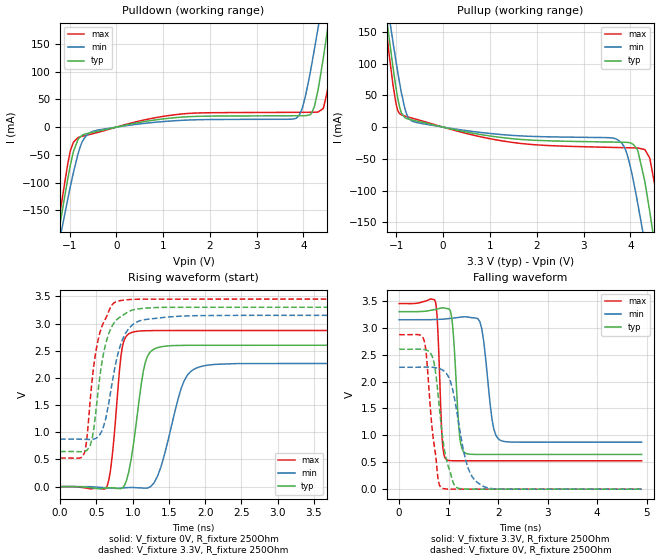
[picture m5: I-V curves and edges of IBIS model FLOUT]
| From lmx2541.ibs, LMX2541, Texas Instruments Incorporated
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|   Model FLOUT
[Model]   FLOUT
Model_type   Output
Polarity   Non-Inverting
Vmeas = 1.65
Vref = 3.3
Cref = 1pF
Rref = 250
|   typ   min   max
|   (nom PVT)   (fast PVT)   (slow PVT)
C_comp   0.475p   0.458p   0.490p
|C_comp (ON state)   0.475p   0.458p   0.490p
|C_comp (OFF state)   0.478p   0.460p   0.493p
[Voltage Range]   3.3   3.15   3.45
[Temperature Range]   27   125   -40
[Pullup Reference]   3.3   3.15   3.45
[Pulldown Reference]   0   0   0
[Power Clamp Reference]   3.3   3.15   3.45
[GND Clamp Reference]   0   0   0
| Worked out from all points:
|   slope of the pulldown table from 0 to 0.495 V, typ, clamps not added: 58.3 ohm
|   slope of the pullup table from 0 to 0.495 V, typ, clamps not added: 64.6 ohm
|   falling waveform, V_fixture 3.3V, R_fixture 250Ohm: 20-80 % time 101ps typ, 157ps min, 72ps max; typ from 3.3 V to 0.646 V
|   rising waveform, V_fixture 0V, R_fixture 250Ohm: 20-80 % time 161ps typ, 262ps min, 111ps max; typ from 0 V to 2.6 V
|   rising waveform, V_fixture 3.3V, R_fixture 250Ohm: 20-80 % time 185ps typ, 217ps min, 171ps max; typ from 0.646 V to 3.3 V
|   falling waveform, V_fixture 0V, R_fixture 250Ohm: 20-80 % time 215ps typ, 282ps min, 176ps max; typ from 2.6 V to 0 V
[Pulldown]
|   Voltage   I(typ)   I(min)   I(max)
-3.3V     -1.312A    -1.152A    -1.46A
-1.253V   -200mA     -221.6mA   -183.3mA
-1.204V   -174.5mA   -200.1mA   -154.2mA
-916.6mV  -43.87mA   -81.81mA   -27.25mA
-530.5mV  -9.772mA   -8.463mA   -12.43mA
3.845V    20.45mA    16.17mA    26.65mA
4.033V    20.59mA    52.73mA    26.74mA
4.311V    66.34mA    177.9mA    27.13mA
4.548V    196.6mA    298.2mA    85.22mA
4.627V    244mA      339.1mA    131.4mA
4.895V    407.4mA    478.8mA    313.3mA
6.598V    1.48A      1.389A     1.531A
[Pullup]
|   Voltage   I(typ)   I(min)   I(max)
-3.3V     1.483A     1.311A     1.641A
-1.223V   180.9mA    208.6mA    160mA
-1.154V   140.4mA    174mA      114.4mA
-896.8mV  22.87mA    55.52mA    19.43mA
-639.4mV  10.9mA     8.688mA    13.73mA
3.697V    -23.67mA   -18.69mA   -32.1mA
3.915V    -23.98mA   -39.26mA   -32.46mA
4.132V    -33.26mA   -110.3mA   -32.83mA
4.311V    -86.09mA   -183.5mA   -35.42mA
4.519V    -184.7mA   -273.9mA   -89.75mA
4.677V    -267.2mA   -344.2mA   -173.2mA
6.598V    -1.311A    -1.221A    -1.366A
[Ramp]
R_load = 250
|   typ   min   max
dV/dt_r   1.56044/1.60576e-10   1.3598/2.61637e-10   1.72318/1.11362e-10
dV/dt_f   1.59265/1.00822e-10   1.36599/1.565e-10   1.75366/7.20184e-11
[Falling Waveform]
V_fixture = 3.3V
V_fixture_min = 3.15V
V_fixture_max = 3.45V
R_fixture = 250Ohm
C_fixture = 0F
|   Time   V(typ)   V(min)   V(max)
0s        3.3V       3.15V      3.45V
737.4ps   3.342V     3.154V     3.472V
872.4ps   3.371V     3.16V      887.7mV
965.6ps   3.358V     3.168V     544.8mV
1.071ns   3.128V     3.177V     528.6mV
1.224ns   971.5mV    3.195V     527.4mV
1.329ns   674.3mV    3.205V     527.4mV
1.631ns   646.2mV    3.114V     527.4mV
2.043ns   646.1mV    909.5mV    527.4mV
4.9ns     645.6mV    873.4mV    527.2mV
[Rising Waveform]
V_fixture = 0V
V_fixture_min = 0V
V_fixture_max = 0V
R_fixture = 250Ohm
C_fixture = 0F
|   Time   V(typ)   V(min)   V(max)
0s        689.3pV    4.847nV    566pV
647.9ps   -23.57mV   -22.39mV   9.795mV
716.6ps   -21.51mV   -28.67mV   543.8mV
838.1ps   -34.97mV   -26.98mV   2.399V
965.6ps   408mV      -16.63mV   2.824V
1.148ns   2.131V     -26.52mV   2.867V
1.329ns   2.55V      156.9mV    2.871V
1.668ns   2.597V     1.803V     2.871V
1.876ns   2.6V       2.179V     2.872V
4.9ns     2.601V     2.266V     2.872V
[Rising Waveform]
V_fixture = 3.3V
V_fixture_min = 3.15V
V_fixture_max = 3.45V
R_fixture = 250Ohm
C_fixture = 0F
|   Time   V(typ)   V(min)   V(max)
0s        645.6mV    873.4mV    527.2mV
317.8ps   644.8mV    870.7mV    573.6mV
365.1ps   664.8mV    868.7mV    843.4mV
411.6ps   745.4mV    866.9mV    1.542V
534.5ps   1.885V     928.6mV    2.763V
640.2ps   2.688V     1.325V     3.127V
767.6ps   3.053V     2.276V     3.399V
910.5ps   3.193V     2.84V      3.435V
1.169ns   3.282V     3.073V     3.449V
4.9ns     3.3V       3.15V      3.45V
[Falling Waveform]
|Gnd
V_fixture = 0V
V_fixture_min = 0V
V_fixture_max = 0V
R_fixture = 250Ohm
C_fixture = 0F
|   Time   V(typ)   V(min)   V(max)
0s        2.601V     2.266V     2.872V
500.6ps   2.597V     2.268V     2.775V
553.3ps   2.585V     2.269V     2.461V
693ps     2.399V     2.264V     913.5mV
784.1ps   1.781V     2.249V     204.9mV
856.9ps   1.126V     2.225V     23.1mV
1.12ns    68.32mV    1.679V     138.5uV
1.391ns   1.004mV    397.5mV    128.5uV
1.668ns   460uV      69.28mV    118.2uV
4.9ns     -30.05uV   -9.735uV   -1.845uV
